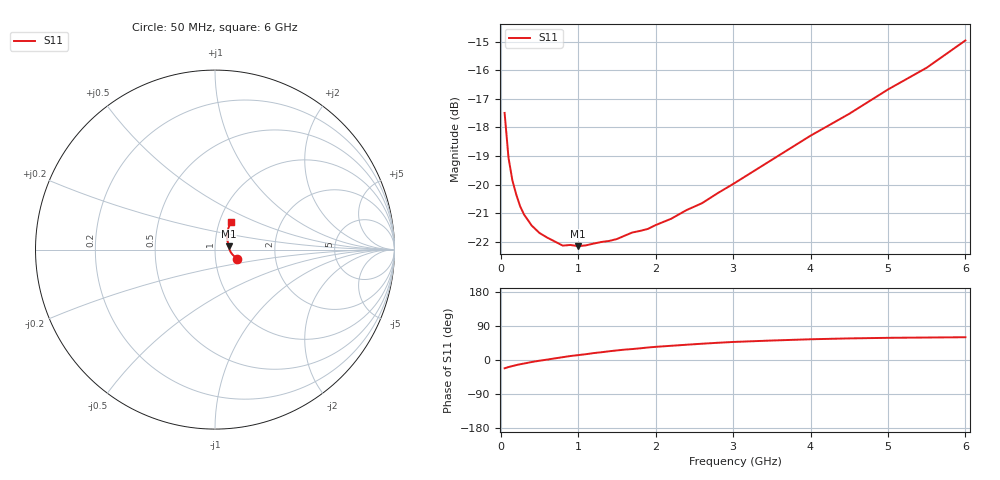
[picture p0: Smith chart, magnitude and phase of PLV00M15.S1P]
! Infineon Technologies  Discrete & RF Semiconductors
! BAR 64-04W /-05W /-06W
! Si PIN Diode in SOT323
! IF = 0.15 mA
! S-Parameters:  October  2008
# GHz  S  MA  R  50
!  f  S11
! GHz  MAG  ANG
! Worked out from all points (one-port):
!   34 points, 50 MHz to 6 GHz, reference 50 ohm
!   lowest |S11| = -22.2 dB at 1 GHz (marker M1), VSWR 1.17, Z = 58.2 + j2.04 ohm
!   |S11| at or under -10 dB: start of sweep to end of sweep
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0.05  0.1334 -21.9
0.1  0.1115 -18.6
0.15  0.1017 -16.0
0.2  0.09607 -13.5
0.25  0.09164 -11.2
0.3  0.08866 -9.4
0.4  0.08475 -5.3
0.5  0.08227 -1.9
0.8  0.07819 7.4
0.9  0.07839 10.5
1  0.07801 12.9
1.1  0.07827 15.3
1.3  0.07934 20.5
1.4  0.07967 23.0
1.5  0.08029 25.3
1.6  0.08137 27.4
1.7  0.08243 28.9
1.9  0.08363 33.0
2  0.08493 34.7
2.2  0.08711 37.5
2.4  0.09023 40.3
2.6  0.09277 43.0
3.5  0.1105 51.4
4  0.1217 54.7
4.5  0.133 57.0
5  0.1467 58.5
5.5  0.1601 59.3
6  0.1787 60.1
